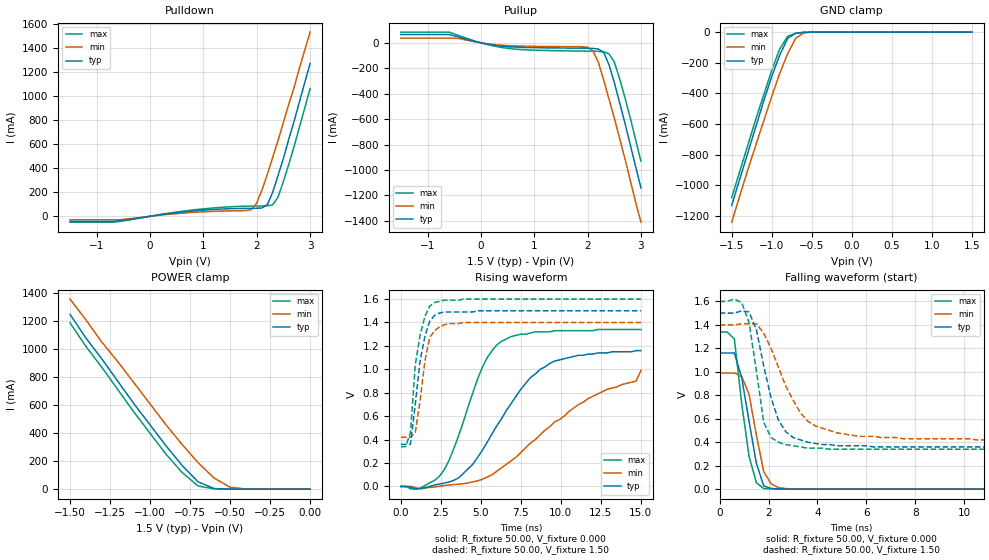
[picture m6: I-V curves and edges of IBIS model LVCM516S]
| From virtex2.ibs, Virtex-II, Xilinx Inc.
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|   Model LVCM516S
[Model]   LVCM516S
Model_type   I/O
Polarity   Non-Inverting
Enable   Active-Low
Vinh = 1.05V
Vinl = 0.3V
Vmeas =   0.75V
Cref =  0pF
Rref =   1.00M
Vref =  0.000V
C_comp   10.00pF   10.00pF   10.00pF
[Temperature Range]   25.00   100.00   0.000
[Voltage Range]   1.50V   1.40V   1.60V
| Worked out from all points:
|   slope of the pulldown table from 0 to 0.225 V, typ, clamps not added: 15.1 ohm
|   slope of the pullup table from 0 to 0.225 V, typ, clamps not added: 13.2 ohm
|   GND clamp passes 1 mA (typ) near -0.57 V on its own axis
|   POWER clamp passes 1 mA (typ) near -0.52 V on its own axis
|   rising waveform, R_fixture 50.00, V_fixture 0.000: 20-80 % time 3.38ns typ, 5.65ns min, 2.15ns max; typ from 0 V to 1.16 V
|   rising waveform, R_fixture 50.00, V_fixture 1.50: 20-80 % time 687ps typ, 628ps min, 640ps max; typ from 0.36 V to 1.5 V
|   falling waveform, R_fixture 50.00, V_fixture 0.000: 20-80 % time 572ps typ, 538ps min, 503ps max; typ from 1.16 V to 0 V
|   falling waveform, R_fixture 50.00, V_fixture 1.50: 20-80 % time 821ps typ, 1.35ns min, 532ps max; typ from 1.5 V to 0.36 V
[Pulldown]
| voltage   I(typ)   I(min)   I(max)
-1.5V     -42.67mA   -28.72mA   -48.9mA
-700mV    -42.67mA   -28.72mA   -48.9mA
800mV     43.93mA    32.22mA    52.52mA
1.9V      66.27mA    55.78mA    84.76mA
2V        66.76mA    110mA      85.3mA
2.1V      69.07mA    220mA      85.82mA
2.2V      98.85mA    350mA      87.26mA
2.3V      200mA      490mA      96.52mA
2.4V      340mA      630mA      160mA
2.5V      480mA      780mA      290mA
2.7V      790mA      1.07A      580mA
3V        1.27A      1.53A      1.06A
[Pullup]
| voltage   I(typ)   I(min)   I(max)
-1.5V     65.27mA    36.47mA    84.3mA
-600mV    65.27mA    36.47mA    84.3mA
100mV     -8.32mA    -6.21mA    -11.27mA
600mV     -32.72mA   -23.85mA   -47.93mA
1.9V      -42.19mA   -30.93mA   -64.82mA
2.1V      -43.7mA    -63.33mA   -65.77mA
2.2V      -48.81mA   -150mA     -66.99mA
2.3V      -73.48mA   -290mA     -72.22mA
2.4V      -170mA     -440mA     -85.88mA
2.5V      -310mA     -590mA     -150mA
2.7V      -630mA     -910mA     -430mA
3V        -1.14A     -1.41A     -930mA
[GND_clamp]
| voltage   I(typ)   I(min)   I(max)
-1.5V     -1.13A     -1.24A     -1.08A
-1.3V     -790mA     -900mA     -740mA
-1.2V     -620mA     -740mA     -570mA
-1.1V     -450mA     -580mA     -410mA
-1V       -290mA     -420mA     -250mA
-900mV    -150mA     -270mA     -110mA
-800mV    -40.96mA   -140mA     -27.15mA
-700mV    -7.52mA    -40.16mA   -8.06mA
-600mV    -1.38mA    -5.56mA    -1.57mA
-500mV    -120uA     -650uA     -120uA
1.5V      27.96pA    98.69nA    16.96pA
[POWER_clamp]
| voltage   I(typ)   I(min)   I(max)
-1.5V     1.25A      1.36A      1.19A
-1.4V     1.08A      1.21A      1.02A
-1.3V     930mA      1.05A      870mA
-1.2V     770mA      910mA      710mA
-1.1V     610mA      760mA      550mA
-900mV    310mA      460mA      250mA
-800mV    170mA      320mA      120mA
-700mV    52.75mA    190mA      22.81mA
-600mV    4.57mA     79.88mA    2.44mA
-500mV    270uA      13.45mA    250uA
-400mV    16.38uA    820uA      14.46uA
0V        27.96pA    880pA      24.27pA
[Ramp]
| variable   typ   min   max
dV/dt_r   0.69/3.38n   0.54/4.84n   0.80/2.15n
dV/dt_f   0.68/0.85n   0.59/1.33n   0.76/0.60n
R_load = 50.00
[Rising Waveform]
R_fixture = 50.00
V_fixture = 0.000
| time   V(typ)   V(min)   V(max)
0s        0V         0V         0V
1.2ns     -17.41mV   -21.13mV   -15.31mV
2.7ns     28.3mV     7.31mV     140mV
3.6ns     72.77mV    19.16mV    430mV
5.1ns     310mV      61.46mV    1.02V
6.3ns     580mV      160mV      1.24V
8.1ns     930mV      370mV      1.31V
9.6ns     1.07V      550mV      1.33V
14.7ns    1.16V      900mV      1.34V
15ns      1.16V      990mV      1.34V
[Rising Waveform]
R_fixture = 50.00
V_fixture = 1.50
V_fixture_min = 1.40
V_fixture_max = 1.60
| time   V(typ)   V(min)   V(max)
0s        360mV      420mV      340mV
300ps     360mV      420mV      340mV
600ps     360mV      420mV      460mV
900ps     700mV      460mV      1.04V
1.2ns     1.07V      730mV      1.29V
1.5ns     1.28V      1.07V      1.45V
1.8ns     1.41V      1.27V      1.54V
2.1ns     1.46V      1.33V      1.57V
3.9ns     1.49V      1.4V       1.6V
15ns      1.5V       1.4V       1.6V
[Falling Waveform]
R_fixture = 50.00
V_fixture = 0.000
| time   V(typ)   V(min)   V(max)
0s        1.16V      990mV      1.34V
300ps     1.16V      990mV      1.34V
600ps     1.16V      990mV      1.28V
900ps     950mV      960mV      730mV
1.2ns     580mV      810mV      280mV
1.5ns     220mV      460mV      55.68mV
1.8ns     27.91mV    150mV      4.53mV
2.1ns     6.02mV     45.65mV    2.04mV
2.7ns     1.75mV     4.96mV     1.1mV
15ns      -31.3uV    -20.92uV   19.93uV
[Falling Waveform]
R_fixture = 50.00
V_fixture = 1.50
V_fixture_min = 1.40
V_fixture_max = 1.60
| time   V(typ)   V(min)   V(max)
0s        1.5V       1.4V       1.6V
900ps     1.52V      1.41V      1.59V
1.2ns     1.51V      1.41V      1.42V
1.5ns     1.36V      1.41V      1.01V
1.8ns     1.05V      1.33V      570mV
2.4ns     590mV      1.04V      400mV
3ns       440mV      760mV      370mV
3.6ns     400mV      580mV      350mV
4.8ns     370mV      480mV      340mV
15ns      360mV      420mV      340mV
